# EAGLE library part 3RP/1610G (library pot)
16mm Potentiometer two level Source: http://www.alphapotentiometers.net/html/16mm_pot_2.html
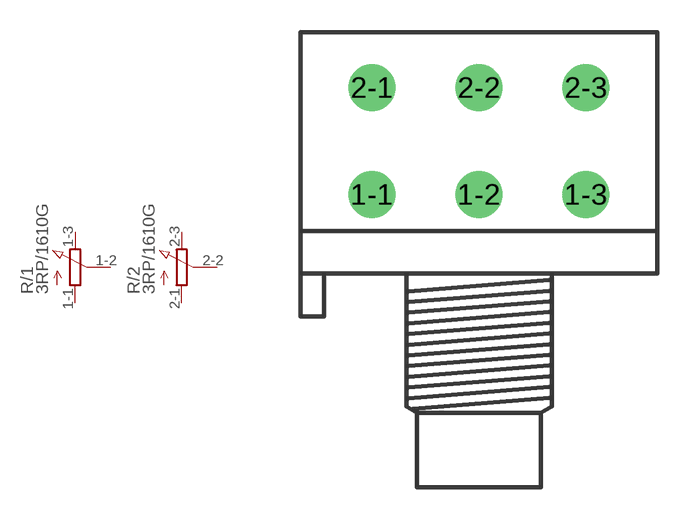
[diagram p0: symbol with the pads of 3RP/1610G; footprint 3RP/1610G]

Designator prefix R; gates /1=POT_EU- /2=POT_EU-

## 3RP/1610G  [3RP/1610G]
1-1  /1:A  pas
1-2  /1:S  pas
1-3  /1:E  pas
2-1  /2:A  pas
2-2  /2:S  pas
2-3  /2:E  pas

## Footprint 3RP/1610G (pad centres in mm)
16mm Potentiometer two level Source: http://www.alphapotentiometers.net/html/16mm_pot_2.html
drill 1.2 pad 2.184: 1-1 -5,0; 1-2 0,0; 1-3 5,0; 2-1 -5,5; 2-2 0,5; 2-3 5,5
